(* Logix 5000 Controller export EFlo_Unidrum_Controller; controller EFlo_Unidrum_Controller 1768-L45 rev 20.12; software revision 20.01 *)

TASK MainTask (continuous, watchdog 500 ms) : MainProgram

MODULES
   Local : 1768-L45 (1768Ctrl5Slot 0, Compact 0, rev 20.12)
      ENET : 1768-ENBT/A (1768 1, Ethernet 10.10.20.11, rev 3.1)
         EFlo_Unidrum : ETHERNET-MODULE (Ethernet 192.168.2.16, rev 1.1, Output RPI 10 ms)   // Graco E-Flo Unidrum
END_MODULES

TYPE ControlBits :
STRUCT
   SystemEnableRequest : BOOL;   // Will enable all the pumps on system
   SystemDisableRequest : BOOL;   // Will disable all the pumps on the system
   PLCControlLockout : BOOL;
   PumpsEnable : BOOL;
   PressureControlEnable : BOOL;
   FlowControlEnable : BOOL;
   AcknowledgeClearErrors : BOOL;
   PrimeRequest : BOOL;   // Applies to the active unit if the active unit is disabled, applies to the inactive unit if the active units is enabled
   DepressurizationRequest : BOOL;
   CrossOverRequest : BOOL;
END_STRUCT
END_TYPE

TYPE DataExchangeStatus :
STRUCT
   DataExchangeCommand : INT; {access Read Only}
   DataExchangeCommandValue : DINT; {access Read Only}
END_STRUCT
END_TYPE

TYPE HeartbeatLogic :
STRUCT
   Failure : BOOL;
   EFloUnidrumDisconnected : BOOL;
   HighMonitor : COUNTER;
   LowMonitor : COUNTER;
   MonitorTimer : TIMER;
   StopMonitorTimer : BOOL;
END_STRUCT
END_TYPE

TYPE PumpsTargets :
STRUCT
   PressureTarget : INT;   // XX.X bar
   FlowTarget : INT;   // XXXX cc/min
END_STRUCT
END_TYPE

TYPE StatusBits :
STRUCT
   Heartbeat : BOOL; {access Read Only}
   AutomationControlReady : BOOL; {access Read Only}
   PLCControlLockoutActive : BOOL; {access Read Only}
   SystemIsEnabled : BOOL; {access Read Only}
   PumpsTryingToMove : BOOL; {access Read Only}
   PumpsIsActuallyMoving : BOOL; {access Read Only}
   NoActiveUnitAlarms : BOOL; {access Read Only}
   NoActiveUnitDeviations : BOOL; {access Read Only}
   NoActiveUnitAdvisories : BOOL; {access Read Only}
   PrimeActive : BOOL; {access Read Only}
   DepressurizationActive : BOOL; {access Read Only}
   DrumLow : BOOL; {access Read Only}
   DrumEmpty : BOOL; {access Read Only}
   PumpNotPrimed : BOOL; {access Read Only}
   DrumNotInPlace : BOOL; {access Read Only}
   PlatenNotInDrum : BOOL; {access Read Only}
   PumpsDisableFromEnclosure : BOOL; {access Read Only}
   Unit1Active : BOOL; {access Read Only}   // For Tandem system only (1 = Unit 1 Active, 0 = Unit 2 Active)
END_STRUCT
END_TYPE

TYPE StatusInformation :
STRUCT
   ActualPumpsFlowrate : INT; {access Read Only}   // XXXX cc/min
   PumpOutletPressure : INT; {access Read Only}   // XX.X bar
   DrumMaterialRemaining : INT; {access Read Only}   // XXX%
END_STRUCT
END_TYPE

TYPE SystemADMInformation :
STRUCT
   CurrentDate : DINT; {access Read Only}   // Bits 0-7 is day Bits 8-15 is month Bits 16-23 is year
   CurrentTime : DINT; {access Read Only}   // Bits 0-7 is seconds Bits 8-15 is minutes Bits 16-23 is hours
   RequestDate : DINT;   // Bits 0-7 is day Bits 8-15 is month Bits 16-23 is year Bit 24 is to trigger ADM process the request
   RequestTime : DINT;   // Bits 0-7 is seconds Bits 8-15 is minutes Bits 16-23 is hours Bit 24 is to trigger ADM process the request
END_STRUCT
END_TYPE

TYPE SystemControlInformation :
STRUCT
   ControlBits : ControlBits;
   PumpTargets : PumpsTargets;   // If Tandem, will only be used for pumps targets. If Ram will be used for targets and priming
   TandemPrimingTargets : PumpsTargets;   // Only used on tandem systems
   DataExchangeCommand : INT;
END_STRUCT
END_TYPE

TYPE UnitStatusInformation :
STRUCT
   StatusBits : StatusBits; {access Read Only}
   Information : StatusInformation; {access Read Only}
   Heartbeat : HeartbeatLogic; {access Read Only}
   DataExchangeStatus : DataExchangeStatus; {access Read Only}
END_STRUCT
END_TYPE

VAR_GLOBAL   (* controller tags *)
   ActiveUnit : UnitStatusInformation := (Heartbeat.HighMonitor.PRE := 2, Heartbeat.LowMonitor.PRE := 2, Heartbeat.MonitorTimer.PRE := 2000); {access Read Only}
   InactiveUnit : UnitStatusInformation := (Heartbeat.HighMonitor.PRE := 2, Heartbeat.LowMonitor.PRE := 2, Heartbeat.MonitorTimer.PRE := 2000); {access Read Only}
   SystemADMInformation : SystemADMInformation;
   SystemControl : SystemControlInformation;
END_VAR

PROGRAM MainProgram   (* main routine MainRoutine *)

ROUTINE EFlo_Unidrum_Data_Mapping   (* ladder *)
// Mapping EFlo Unidrum Data to tags
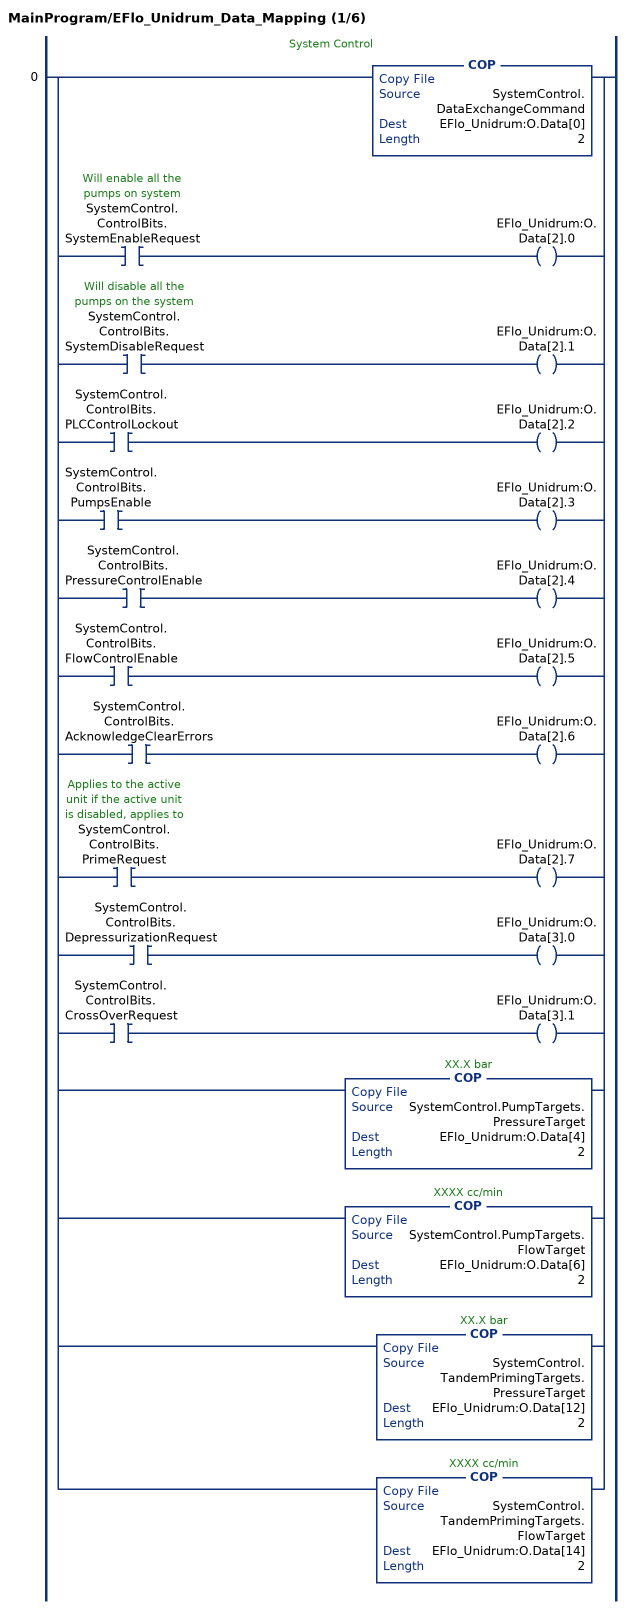
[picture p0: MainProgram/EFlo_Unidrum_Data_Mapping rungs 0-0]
   // System Control
   0: [COP(SystemControl.DataExchangeCommand,EFlo_Unidrum:O.Data[0],2) ,XIC(SystemControl.ControlBits.SystemEnableRequest) OTE(EFlo_Unidrum:O.Data[2].0) ,XIC(SystemControl.ControlBits.SystemDisableRequest) OTE(EFlo_Unidrum:O.Data[2].1) ,XIC(SystemControl.ControlBits.PLCControlLockout) OTE(EFlo_Unidrum:O.Data[2].2) ,XIC(SystemControl.ControlBits.PumpsEnable) OTE(EFlo_Unidrum:O.Data[2].3) ,XIC(SystemControl.ControlBits.PressureControlEnable) OTE(EFlo_Unidrum:O.Data[2].4) ,XIC(SystemControl.ControlBits.FlowControlEnable) OTE(EFlo_Unidrum:O.Data[2].5) ,XIC(SystemControl.ControlBits.AcknowledgeClearErrors) OTE(EFlo_Unidrum:O.Data[2].6) ,XIC(SystemControl.ControlBits.PrimeRequest) OTE(EFlo_Unidrum:O.Data[2].7) ,XIC(SystemControl.ControlBits.DepressurizationRequest) OTE(EFlo_Unidrum:O.Data[3].0) ,XIC(SystemControl.ControlBits.CrossOverRequest) OTE(EFlo_Unidrum:O.Data[3].1) ,COP(SystemControl.PumpTargets.PressureTarget,EFlo_Unidrum:O.Data[4],2) ,COP(SystemControl.PumpTargets.FlowTarget,EFlo_Unidrum:O.Data[6],2) ,COP(SystemControl.TandemPrimingTargets.PressureTarget,EFlo_Unidrum:O.Data[12],2) ,COP(SystemControl.TandemPrimingTargets.FlowTarget,EFlo_Unidrum:O.Data[14],2) ];
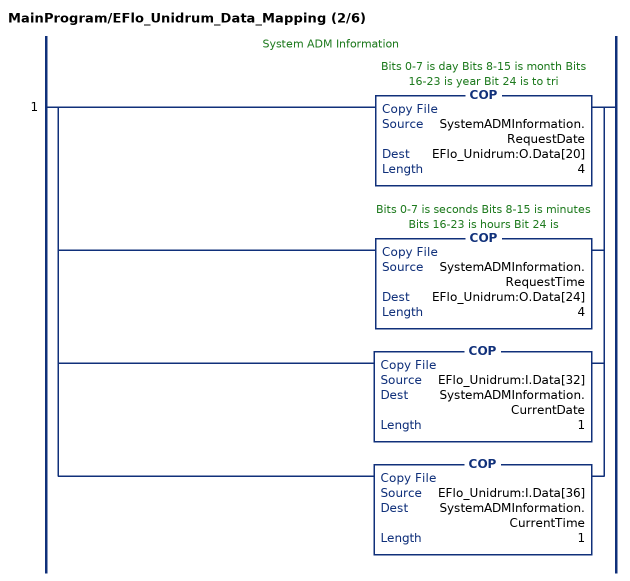
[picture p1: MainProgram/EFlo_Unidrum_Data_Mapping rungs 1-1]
   // System ADM Information
   1: [COP(SystemADMInformation.RequestDate,EFlo_Unidrum:O.Data[20],4) ,COP(SystemADMInformation.RequestTime,EFlo_Unidrum:O.Data[24],4) ,COP(EFlo_Unidrum:I.Data[32],SystemADMInformation.CurrentDate,1) ,COP(EFlo_Unidrum:I.Data[36],SystemADMInformation.CurrentTime,1) ];
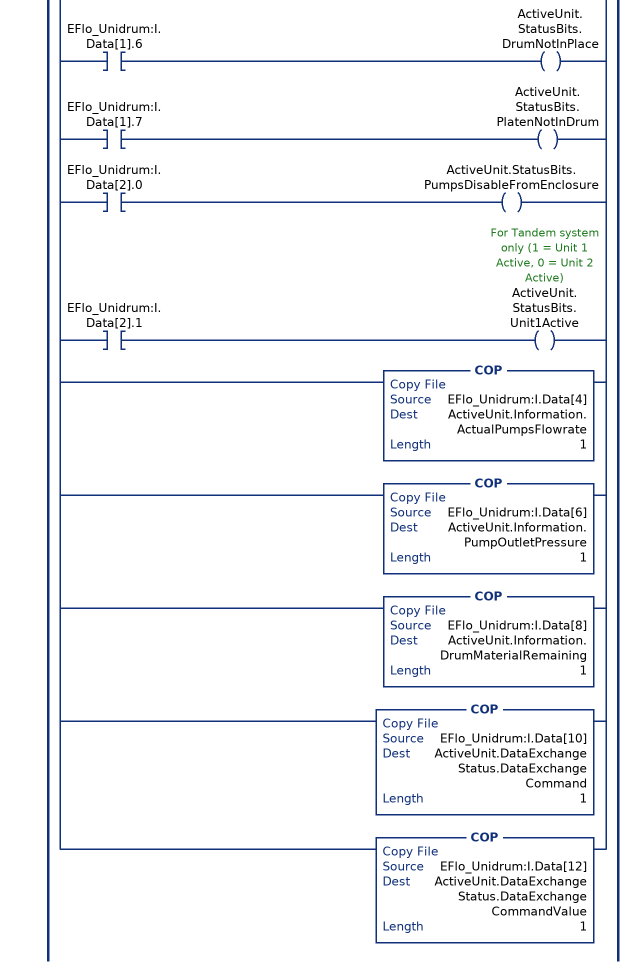
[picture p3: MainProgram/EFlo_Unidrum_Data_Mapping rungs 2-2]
   // Active Unit
   2: [XIC(EFlo_Unidrum:I.Data[0].0) OTE(ActiveUnit.StatusBits.Heartbeat) ,XIC(EFlo_Unidrum:I.Data[0].1) OTE(ActiveUnit.StatusBits.AutomationControlReady) ,XIC(EFlo_Unidrum:I.Data[0].2) OTE(ActiveUnit.StatusBits.PLCControlLockoutActive) ,XIC(EFlo_Unidrum:I.Data[0].3) OTE(ActiveUnit.StatusBits.SystemIsEnabled) ,XIC(EFlo_Unidrum:I.Data[0].4) OTE(ActiveUnit.StatusBits.PumpsTryingToMove) ,XIC(EFlo_Unidrum:I.Data[0].5) OTE(ActiveUnit.StatusBits.PumpsIsActuallyMoving) ,XIC(EFlo_Unidrum:I.Data[0].6) OTE(ActiveUnit.StatusBits.NoActiveUnitAlarms) ,XIC(EFlo_Unidrum:I.Data[0].7) OTE(ActiveUnit.StatusBits.NoActiveUnitDeviations) ,XIC(EFlo_Unidrum:I.Data[1].0) OTE(ActiveUnit.StatusBits.NoActiveUnitAdvisories) ,XIC(EFlo_Unidrum:I.Data[1].1) OTE(ActiveUnit.StatusBits.PrimeActive) ,XIC(EFlo_Unidrum:I.Data[1].2) OTE(ActiveUnit.StatusBits.DepressurizationActive) ,XIC(EFlo_Unidrum:I.Data[1].3) OTE(ActiveUnit.StatusBits.DrumLow) ,XIC(EFlo_Unidrum:I.Data[1].4) OTE(ActiveUnit.StatusBits.DrumEmpty) ,XIC(EFlo_Unidrum:I.Data[1].5) OTE(ActiveUnit.StatusBits.PumpNotPrimed) ,XIC(EFlo_Unidrum:I.Data[1].6) OTE(ActiveUnit.StatusBits.DrumNotInPlace) ,XIC(EFlo_Unidrum:I.Data[1].7) OTE(ActiveUnit.StatusBits.PlatenNotInDrum) ,XIC(EFlo_Unidrum:I.Data[2].0) OTE(ActiveUnit.StatusBits.PumpsDisableFromEnclosure) ,XIC(EFlo_Unidrum:I.Data[2].1) OTE(ActiveUnit.StatusBits.Unit1Active) ,COP(EFlo_Unidrum:I.Data[4],ActiveUnit.Information.ActualPumpsFlowrate,1) ,COP(EFlo_Unidrum:I.Data[6],ActiveUnit.Information.PumpOutletPressure,1) ,COP(EFlo_Unidrum:I.Data[8],ActiveUnit.Information.DrumMaterialRemaining,1) ,COP(EFlo_Unidrum:I.Data[10],ActiveUnit.DataExchangeStatus.DataExchangeCommand,1) ,COP(EFlo_Unidrum:I.Data[12],ActiveUnit.DataExchangeStatus.DataExchangeCommandValue,1) ];
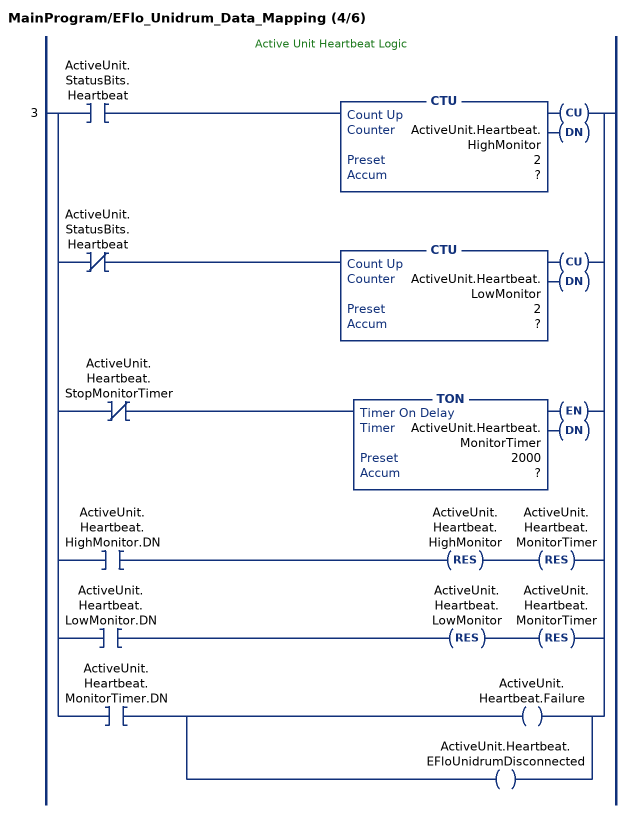
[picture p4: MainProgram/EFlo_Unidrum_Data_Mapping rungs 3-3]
   // Active Unit Heartbeat Logic
   3: [XIC(ActiveUnit.StatusBits.Heartbeat) CTU(ActiveUnit.Heartbeat.HighMonitor,?,?) ,XIO(ActiveUnit.StatusBits.Heartbeat) CTU(ActiveUnit.Heartbeat.LowMonitor,?,?) ,XIO(ActiveUnit.Heartbeat.StopMonitorTimer) TON(ActiveUnit.Heartbeat.MonitorTimer,?,?) ,XIC(ActiveUnit.Heartbeat.HighMonitor.DN) RES(ActiveUnit.Heartbeat.HighMonitor) RES(ActiveUnit.Heartbeat.MonitorTimer) ,XIC(ActiveUnit.Heartbeat.LowMonitor.DN) RES(ActiveUnit.Heartbeat.LowMonitor) RES(ActiveUnit.Heartbeat.MonitorTimer) ,XIC(ActiveUnit.Heartbeat.MonitorTimer.DN) [OTE(ActiveUnit.Heartbeat.Failure) ,OTE(ActiveUnit.Heartbeat.EFloUnidrumDisconnected) ] ];
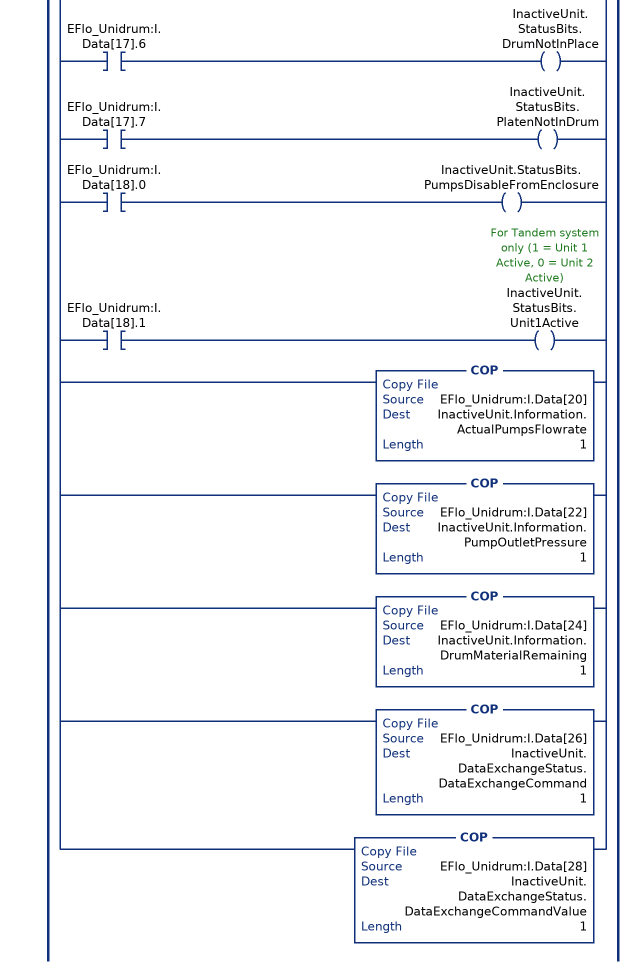
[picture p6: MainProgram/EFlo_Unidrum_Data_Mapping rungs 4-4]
   // Inactive Unit
   4: [XIC(EFlo_Unidrum:I.Data[16].0) OTE(InactiveUnit.StatusBits.Heartbeat) ,XIC(EFlo_Unidrum:I.Data[16].1) OTE(InactiveUnit.StatusBits.AutomationControlReady) ,XIC(EFlo_Unidrum:I.Data[16].2) OTE(InactiveUnit.StatusBits.PLCControlLockoutActive) ,XIC(EFlo_Unidrum:I.Data[16].3) OTE(InactiveUnit.StatusBits.SystemIsEnabled) ,XIC(EFlo_Unidrum:I.Data[16].4) OTE(InactiveUnit.StatusBits.PumpsTryingToMove) ,XIC(EFlo_Unidrum:I.Data[16].5) OTE(InactiveUnit.StatusBits.PumpsIsActuallyMoving) ,XIC(EFlo_Unidrum:I.Data[16].6) OTE(InactiveUnit.StatusBits.NoActiveUnitAlarms) ,XIC(EFlo_Unidrum:I.Data[16].7) OTE(InactiveUnit.StatusBits.NoActiveUnitDeviations) ,XIC(EFlo_Unidrum:I.Data[17].0) OTE(InactiveUnit.StatusBits.NoActiveUnitAdvisories) ,XIC(EFlo_Unidrum:I.Data[17].1) OTE(InactiveUnit.StatusBits.PrimeActive) ,XIC(EFlo_Unidrum:I.Data[17].2) OTE(InactiveUnit.StatusBits.DepressurizationActive) ,XIC(EFlo_Unidrum:I.Data[17].3) OTE(InactiveUnit.StatusBits.DrumLow) ,XIC(EFlo_Unidrum:I.Data[17].4) OTE(InactiveUnit.StatusBits.DrumEmpty) ,XIC(EFlo_Unidrum:I.Data[17].5) OTE(InactiveUnit.StatusBits.PumpNotPrimed) ,XIC(EFlo_Unidrum:I.Data[17].6) OTE(InactiveUnit.StatusBits.DrumNotInPlace) ,XIC(EFlo_Unidrum:I.Data[17].7) OTE(InactiveUnit.StatusBits.PlatenNotInDrum) ,XIC(EFlo_Unidrum:I.Data[18].0) OTE(InactiveUnit.StatusBits.PumpsDisableFromEnclosure) ,XIC(EFlo_Unidrum:I.Data[18].1) OTE(InactiveUnit.StatusBits.Unit1Active) ,COP(EFlo_Unidrum:I.Data[20],InactiveUnit.Information.ActualPumpsFlowrate,1) ,COP(EFlo_Unidrum:I.Data[22],InactiveUnit.Information.PumpOutletPressure,1) ,COP(EFlo_Unidrum:I.Data[24],InactiveUnit.Information.DrumMaterialRemaining,1) ,COP(EFlo_Unidrum:I.Data[26],InactiveUnit.DataExchangeStatus.DataExchangeCommand,1) ,COP(EFlo_Unidrum:I.Data[28],InactiveUnit.DataExchangeStatus.DataExchangeCommandValue,1) ];
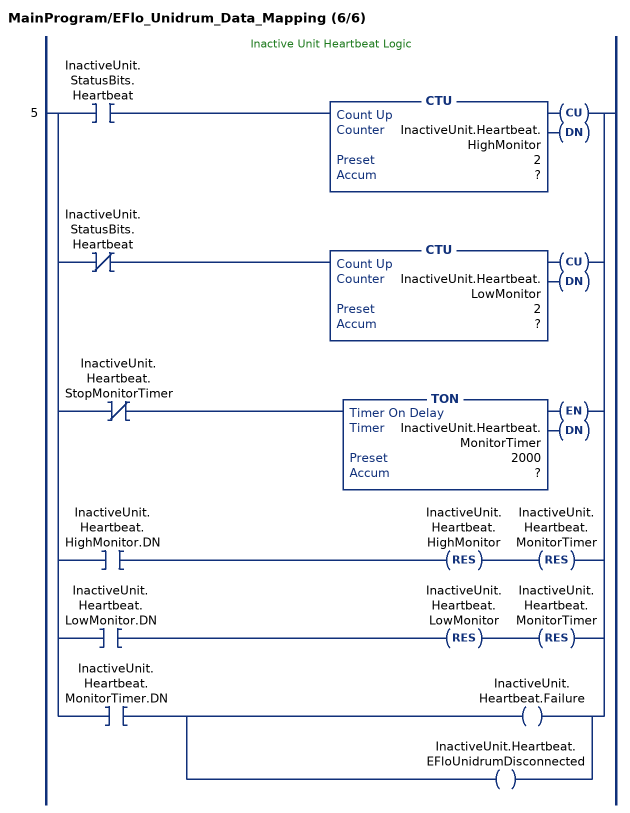
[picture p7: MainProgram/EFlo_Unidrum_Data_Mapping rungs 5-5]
   // Inactive Unit Heartbeat Logic
   5: [XIC(InactiveUnit.StatusBits.Heartbeat) CTU(InactiveUnit.Heartbeat.HighMonitor,?,?) ,XIO(InactiveUnit.StatusBits.Heartbeat) CTU(InactiveUnit.Heartbeat.LowMonitor,?,?) ,XIO(InactiveUnit.Heartbeat.StopMonitorTimer) TON(InactiveUnit.Heartbeat.MonitorTimer,?,?) ,XIC(InactiveUnit.Heartbeat.HighMonitor.DN) RES(InactiveUnit.Heartbeat.HighMonitor) RES(InactiveUnit.Heartbeat.MonitorTimer) ,XIC(InactiveUnit.Heartbeat.LowMonitor.DN) RES(InactiveUnit.Heartbeat.LowMonitor) RES(InactiveUnit.Heartbeat.MonitorTimer) ,XIC(InactiveUnit.Heartbeat.MonitorTimer.DN) [OTE(InactiveUnit.Heartbeat.Failure) ,OTE(InactiveUnit.Heartbeat.EFloUnidrumDisconnected) ] ];
END_ROUTINE

ROUTINE MainRoutine   (* ladder *)
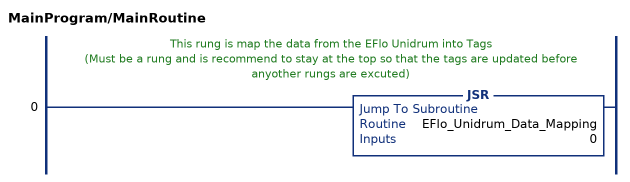
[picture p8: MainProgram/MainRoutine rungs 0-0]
   // This rung is map the data from the EFlo Unidrum into Tags
   // (Must be a rung and is recommend to stay at the top so that the tags are updated before anyother rungs are excuted)
   0: JSR(EFlo_Unidrum_Data_Mapping,0);
END_ROUTINE
END_PROGRAM
